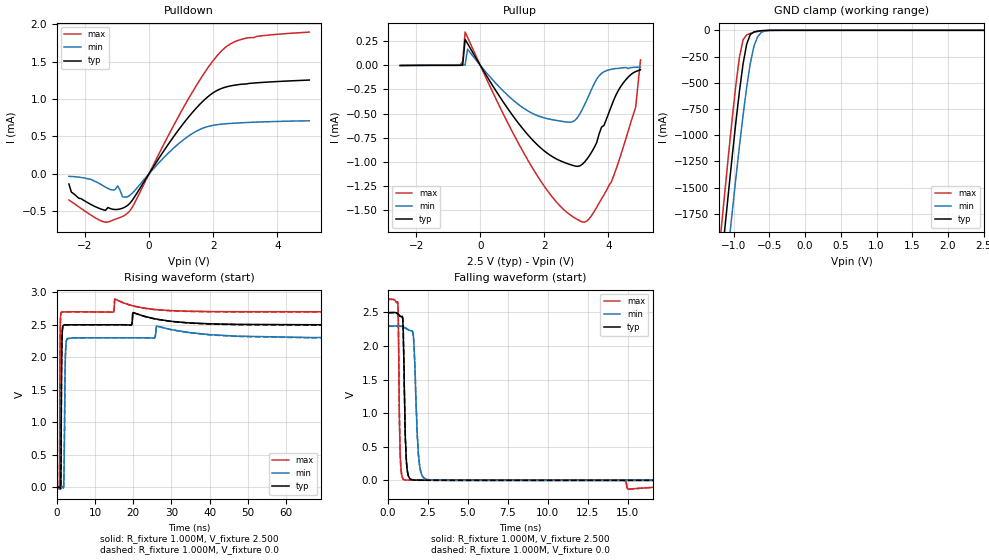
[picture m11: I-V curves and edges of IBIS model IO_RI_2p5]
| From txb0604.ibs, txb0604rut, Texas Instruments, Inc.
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|   Model IO_RI_2p5
[Model] IO_RI_2p5
Model_type 3-state
Polarity   Non-Inverting
Enable   Active-High
Vmeas =  1.250V
Cref =  0.100nF
Rref =  1.000M
Vref =  0.0V
C_comp   3.670pF   3.390pF   3.920pF
[Temperature Range]   27.000   0.125k   -40.000
[Voltage Range]   2.500V   2.300V   2.700V
[Pullup Reference]   2.500V   2.300V   2.700V
[Pulldown Reference]   0.0V   0.0V   0.0V
[POWER Clamp Reference]   2.500V   2.300V   2.700V
[GND Clamp Reference]   0.0V   0.0V   0.0V
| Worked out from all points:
|   slope of the pulldown table from 0 to 0.375 V, typ, clamps not added: 1.49 kohm
|   slope of the pullup table from 0 to 0.375 V, typ, clamps not added: 1.83 kohm
|   GND clamp passes 1 mA (typ) near -0.54 V on its own axis
|   rising waveform, R_fixture 1.000M, V_fixture 2.500: 20-80 % time 162ps typ, 248ps min, 112ps max; typ from 0.004 V to 2.5 V
|   rising waveform, R_fixture 1.000M, V_fixture 0.0: 20-80 % time 162ps typ, 247ps min, 112ps max; typ from 0 V to 2.5 V
|   falling waveform, R_fixture 1.000M, V_fixture 2.500: 20-80 % time 139ps typ, 228ps min, 89ps max; typ from 2.5 V to 0.004 V
|   falling waveform, R_fixture 1.000M, V_fixture 0.0: 20-80 % time 140ps typ, 228ps min, 89.2ps max; typ from 2.5 V to 0 V
[Pulldown]
|Voltage   I(typ)   I(min)   I(max)
-2.5V     -137.5uA   -34.69uA   -350.8uA
-2.424V   -246.2uA   -36.54uA   -373.5uA
-2.196V   -327.1uA   -45.09uA   -442.4uA
-1.436V   -481.6uA   -159.8uA   -641.3uA
-1.132V   -475.6uA   -219.1uA   -622.1uA
-980mV    -477.6uA   -162.1uA   -597.9uA
-752mV    -447uA     -313.7uA   -554.2uA
-524mV    -355.9uA   -261.7uA   -449.7uA
1.148V    714.7uA    479uA      943.1uA
2.288V    1.147mA    665.4uA    1.656mA
3.048V    1.204mA    686.3uA    1.817mA
5V        1.255mA    708.9uA    1.898mA
[Pullup]
|Voltage   I(typ)   I(min)   I(max)
-2.5V     -1.764uA   -3.605uA   -1.014uA
-624mV    144.1nA    16.02nA    2.229uA
-548mV    5.189uA    154.5nA    41.4uA
-472mV    267.9uA    4.357uA    344.4uA
-396mV    225.5uA    167.3uA    290.2uA
1.656V    -782.2uA   -503uA     -1.078mA
2.872V    -1.036mA   -586.1uA   -1.566mA
3.252V    -1.003mA   -410.5uA   -1.626mA
3.708V    -710.9uA   -108.3uA   -1.426mA
4.24V     -303.5uA   -32.78uA   -1.074mA
4.848V    -64.71uA   -20.12uA   -436.4uA
5V        -46.3uA    -19.04uA   56.16uA
[GND_clamp]
|Voltage   I(typ)   I(min)   I(max)
-2.5V     -11.36A    -11.16A    -11.58A
-1.174V   -2.242A    -2.754A    -1.903A
-1.123V   -1.891A    -2.412A    -1.543A
-1.072V   -1.546A    -2.075A    -1.19A
-1.021V   -1.21A     -1.743A    -850mA
-919mV    -584.2mA   -1.108A    -257.8mA
-868mV    -320.7mA   -811.8mA   -90.35mA
-817mV    -130.7mA   -541.5mA   -43.06mA
-715mV    -15mA      -149.4mA   -19.5mA
-664mV    -7.355mA   -60.49mA   -11.8mA
-562mV    -1.371mA   -6.057mA   -2.317mA
2.5V      0A         0A         0A
[Ramp]
| variable   typ   min   max
dV/dt_r   1.497/0.162n   1.377/0.243n   1.618/0.117n
dV/dt_f   1.498/0.132n   1.377/0.226n   1.618/89.508p
R_load = 1.000M
[Rising Waveform]
R_fixture= 1.000M
V_fixture= 2.500
V_fixture_min= 2.300
V_fixture_max= 2.700
|time   V(typ)   V(min)   V(max)
0s        3.625mV    4.618mV    3.076mV
650ps     4.364mV    4.334mV    -14.87mV
840ps     4.783mV    3.41mV     2.218V
1ns       -7.454mV   3.488mV    2.649V
1.22ns    1.782V     7.522mV    2.695V
1.41ns    2.399V     8.515mV    2.697V
1.83ns    2.496V     109.2mV    2.698V
2.21ns    2.498V     1.972V     2.699V
2.69ns    2.499V     2.285V     2.699V
120ns     2.5V       2.3V       2.7V
[Rising Waveform]
R_fixture= 1.000M
V_fixture= 0.0
V_fixture_min= 0.0
V_fixture_max= 0.0
|time   V(typ)   V(min)   V(max)
0s        -3.324uV   9.977uV    -4.059uV
650ps     643.4uV    -273.6uV   -18.04mV
840ps     1.05mV     -1.219mV   2.217V
1ns       -11.3mV    -1.211mV   2.649V
1.22ns    1.78V      2.722mV    2.695V
1.41ns    2.399V     3.617mV    2.697V
1.83ns    2.496V     105.2mV    2.698V
2.21ns    2.498V     1.971V     2.699V
2.69ns    2.499V     2.285V     2.699V
120ns     2.496V     2.294V     2.696V
[Falling Waveform]
R_fixture= 1.000M
V_fixture= 2.500
V_fixture_min= 2.300
V_fixture_max= 2.700
|time   V(typ)   V(min)   V(max)
0s        2.5V       2.3V       2.7V
610ps     2.481V     2.301V     2.633V
750ps     2.448V     2.3V       443.8mV
920ps     2.402V     2.29V      28.12mV
1.09ns    568.2mV    2.27V      5.001mV
1.59ns    4.863mV    2.134V     2.015mV
1.82ns    2.716mV    698.3mV    1.615mV
2.01ns    2.166mV    164.9mV    1.413mV
2.78ns    1.216mV    3.461mV    605.2uV
120ns     3.636mV    4.609mV    3.084mV
[Falling Waveform]
R_fixture= 1.000M
V_fixture= 0.0
V_fixture_min= 0.0
V_fixture_max= 0.0
|time   V(typ)   V(min)   V(max)
0s        2.496V     2.294V     2.696V
610ps     2.476V     2.295V     2.63V
750ps     2.443V     2.294V     443.7mV
920ps     2.397V     2.284V     28.03mV
1.09ns    566.5mV    2.265V     4.956mV
1.59ns    4.806mV    2.128V     1.975mV
1.82ns    2.665mV    695.4mV    1.573mV
2.01ns    2.116mV    164.1mV    1.376mV
2.78ns    1.167mV    3.388mV    567.5uV
120ns     7.153uV    1.822uV    5.042uV
